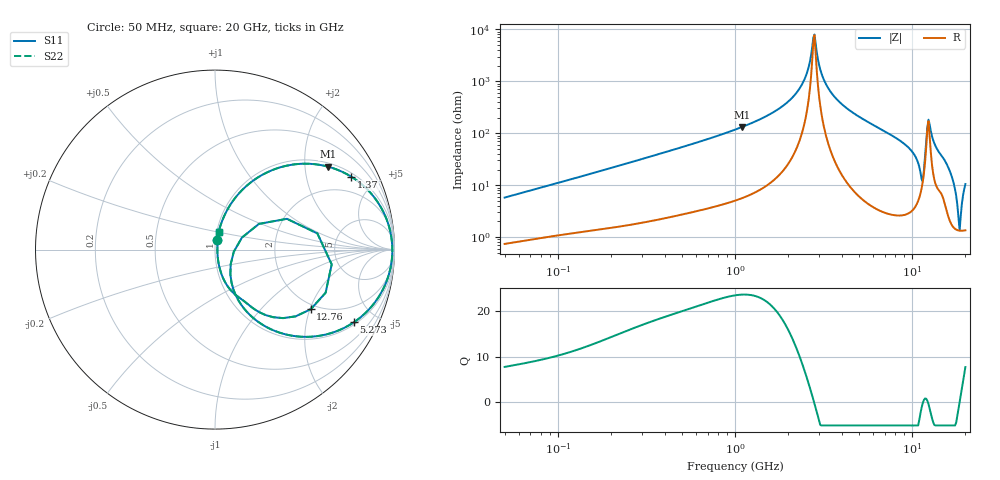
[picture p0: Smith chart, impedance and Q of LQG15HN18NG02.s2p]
!Murata Part Number: LQG15HN18NG02
!These Parameters are Measured in Series Mode Connection
!  o--[Z]--o
!Port1  Port2
!  o-------o
!Freq. Start=50[MHz] Stop=20[GHz], 401[Steps]
# Hz S RI R 50
!Freq.(Hz) S11(Real) S11(Imag) S21(Real) S21(Imag) S12(Real) S12(Imag) S22(Real) S22(Imag)
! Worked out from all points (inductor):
!   401 points, 50 MHz to 20 GHz, reference 50 ohm
!   read as one part in series: L = 17.9 nH near 51.52 MHz
!   highest Q = 23.5 at 1.094 GHz (marker M1), where L = 19.1 nH
!   self-resonance near 2.769 GHz
!   S11 on the Smith chart (normalised r, x): 50 MHz: 1.01, +0.11; 1.37 GHz: 1.16, +3.65; 5.273 GHz: 1.10, -3.75; 12.76 GHz: 1.84, -2.03; 20 GHz: 1.03, +0.21
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5e7  0.0105 0.056  0.9895 -0.056  0.9895 -0.056  0.0105 0.056
1.364002e8  0.0329 0.1411  0.9671 -0.1411  0.9671 -0.1411  0.0329 0.1411
3.721004e8  0.1496 0.3302  0.8504 -0.3302  0.8504 -0.3302  0.1496 0.3302
1e9  0.575 0.4734  0.425 -0.4734  0.425 -0.4734  0.575 0.4734
1.094034e9  0.6287 0.4624  0.3713 -0.4624  0.3713 -0.4624  0.6287 0.4624
1.369645e9  0.7595 0.4061  0.2405 -0.4061  0.2405 -0.4061  0.7595 0.4061
2.245319e9  0.9626 0.151  0.0374 -0.151  0.0374 -0.151  0.9626 0.151
2.531158e9  0.9823 0.0703  0.0177 -0.0703  0.0177 -0.0703  0.9823 0.0703
2.728004e9  0.9875 0.0181  0.0125 -0.0181  0.0125 -0.0181  0.9875 0.0181
2.853386e9  0.9879 -0.0136  0.0121 0.0136  0.0121 0.0136  0.9879 -0.0136
3.075291e9  0.9838 -0.0668  0.0162 0.0668  0.0162 0.0668  0.9838 -0.0668
3.466789e9  0.9648 -0.1514  0.0352 0.1514  0.0352 0.1514  0.9648 -0.1514
5.273168e9  0.7728 -0.4054  0.2272 0.4054  0.2272 0.4054  0.7728 -0.4054
7.442007e9  0.4837 -0.4857  0.5163 0.4857  0.5163 0.4857  0.4837 -0.4857
9.892087e9  0.1931 -0.3626  0.8069 0.3626  0.8069 0.3626  0.1931 -0.3626
1.131968e10  0.0873 -0.0819  0.9127 0.0819  0.9127 0.0819  0.0873 -0.0819
1.201863e10  0.4007 0.1715  0.5993 -0.1715  0.5993 -0.1715  0.4007 0.1715
1.276073e10  0.5334 -0.3323  0.4666 0.3323  0.4666 0.3323  0.5334 -0.3323
1.375312e10  0.2467 -0.3487  0.7533 0.3487  0.7533 0.3487  0.2467 -0.3487
1.621653e10  0.0563 -0.1816  0.9437 0.1816  0.9437 0.1816  0.0563 -0.1816
1.855685e10  0.0131 0.00177  0.9869 -0.00177  0.9869 -0.00177  0.0131 0.00177
2e10  0.0236 0.1001  0.9764 -0.1001  0.9764 -0.1001  0.0236 0.1001
